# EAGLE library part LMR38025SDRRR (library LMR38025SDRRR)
Functional Safety-Capable Documentation available to aid functional safety system design Configured for rugged industrial applications 4.2V to 80V input voltage range 2.5A continuous output current Ultra-low 40A operating quiescent current 200kHz to 2.2MHz adjustable switching frequency Frequency synchronization to external clock 97% maximum duty cycle Supports start-up events with prebiased output +/-1.5% reference voltage tolerance over temperature Precision enable Source: Datasheet
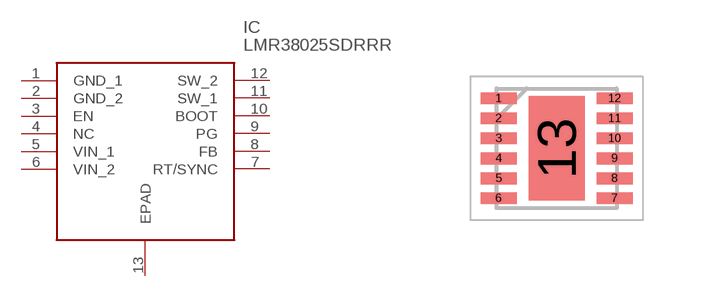
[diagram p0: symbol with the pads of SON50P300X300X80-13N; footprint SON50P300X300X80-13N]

Designator prefix IC

## LMR38025SDRRR (Description: Functional Safety-Capable Documentation available to aid functional safety system design Configured for rugged industrial applications 4.2V to 80V input voltage range 2.5A continuous output current Ultra-low 40A operating quiescent current 200kHz to 2.2MHz adjustable switching frequency Frequency synchronization to external clock 97% maximum duty cycle Supports start-up events with prebiased output +/-1.5% reference voltage tolerance over temperature Precision enable; Height: 0.8mm; Manufacturer_Name: Texas Instruments; Manufacturer_Part_Number: LMR38025SDRRR; Mouser_Part_Number: 595-LMR38025SDRRR; Mouser_Price-Stock: https://www.mouser.co.uk/ProductDetail/Texas-Instruments/LMR38025SDRRR?qs=dbcCsuKDzFX4%252BlLpuICnYw%3D%3D)  [SON50P300X300X80-13N]
1  GND_1
2  GND_2
3  EN
4  NC  nc
5  VIN_1
6  VIN_2
7  RT/SYNC
8  FB
9  PG
10  BOOT
11  SW_1
12  SW_2
13  EPAD

## Footprint SON50P300X300X80-13N (pad centres in mm)
LMR38025SDRRR
smd 0.9 x 0.3: 1 -1.45,1.25; 2 -1.45,0.75; 3 -1.45,0.25; 4 -1.45,-0.25; 5 -1.45,-0.75; 6 -1.45,-1.25; 7 1.45,-1.25; 8 1.45,-0.75; 9 1.45,-0.25; 10 1.45,0.25; 11 1.45,0.75; 12 1.45,1.25
smd 1.4 x 2.6: 13 0,0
